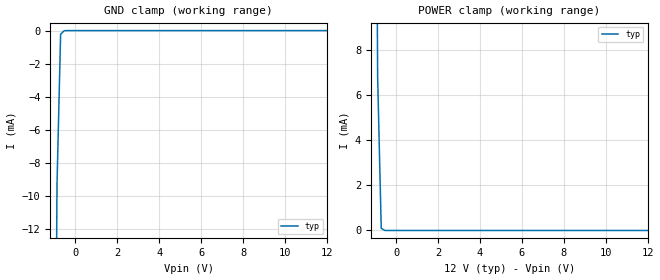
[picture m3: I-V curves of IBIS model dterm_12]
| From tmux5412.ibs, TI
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| dterm_12
[Model]   dterm_12
Model_type   Terminator
|   typ   min   max
C_comp   1.008417e-11   NA   NA
[Voltage Range]   12   NA   NA
[Temperature Range]   27   NA   NA
[Power Clamp Reference]   12   NA   NA
[GND Clamp Reference]   0   NA   NA
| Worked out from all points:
|   GND clamp passes 1 mA (typ) near -0.72 V on its own axis
|   POWER clamp passes 1 mA (typ) near -0.73 V on its own axis
[GND Clamp]
|   Voltage   I(typ)   I(min)   I(max)
-5V       -2.839A    NA         NA
-1.051V   -42.72mA   NA         NA
-878.8mV  -9.288mA   NA         NA
-707.1mV  -223.6uA   NA         NA
-535.4mV  -9.048uA   NA         NA
12V       1.089nA    NA         NA
[POWER Clamp]
|   Voltage   I(typ)   I(min)   I(max)
-5V       2.584A     NA         NA
-1.05V    36.24mA    NA         NA
-878.8mV  6.83mA     NA         NA
-707.1mV  98.83uA    NA         NA
-535.4mV  993nA      NA         NA
12V       -527.7pA   NA         NA
